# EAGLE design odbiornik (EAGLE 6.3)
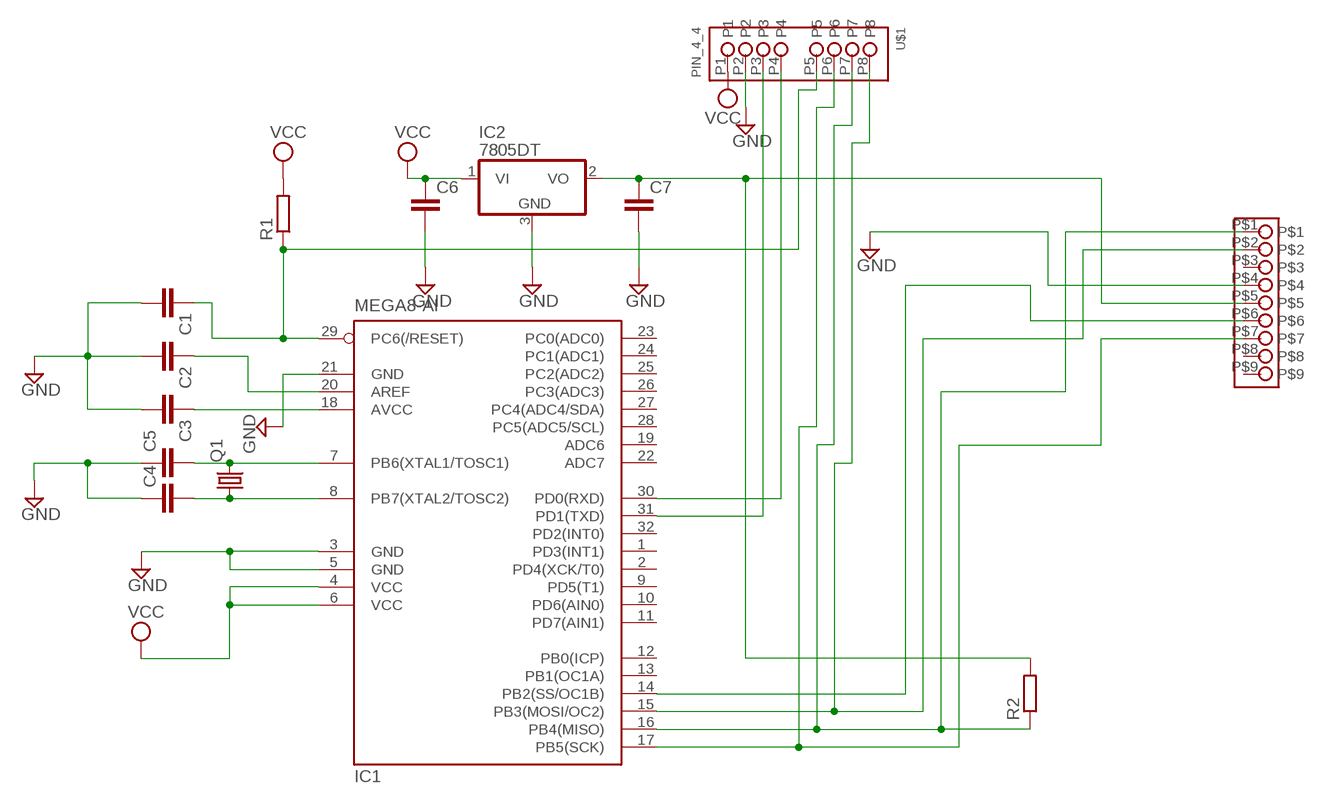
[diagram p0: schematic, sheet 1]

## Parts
C1  C-EUC0805  [C0805]
C2  C-EUC0805  [C0805]
C3  C-EUC0805  [C0805]
C4  C-EUC0805  [C0805]
C5  C-EUC0805  [C0805]
C6  C-EUC0805  [C0805]
C7  C-EUC0805  [C0805]
IC1  MEGA8-AI  [TQFP32-08]
IC2  7805DT  [TO252]
Q1  CRYSTALHC49UP  [HC49UP]
R1  R-EU_M0805  [M0805]
R2  R-EU_R0805  [R0805]
U$1  PIN_4_4  [PIN_4_4]
U$2  PIN_4MM  [PIN_4MM]

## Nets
GND: C1.2 C2.2 C3.2 C4.1 C5.1 C6.2 C7.2 IC1.3(GND) IC1.5(GND) IC1.21(GND) IC2.3(GND) U$1.P2 U$2.P$4
N$1: C3.1 IC1.18(AVCC)
N$2: C2.1 IC1.20(AREF)
N$3: C1.1 IC1.29(PC6(/RESET)) R1.1 U$1.P5
N$4: C5.2 IC1.7(PB6(XTAL1/TOSC1)) Q1.2
N$5: C4.2 IC1.8(PB7(XTAL2/TOSC2)) Q1.1
N$6: IC1.17(PB5(SCK)) U$1.P6 U$2.P$7
N$7: IC1.16(PB4(MISO)) R2.1 U$1.P7 U$2.P$1
N$8: IC1.15(PB3(MOSI/OC2)) U$1.P8 U$2.P$2
N$9: IC1.14(PB2(SS/OC1B)) U$2.P$6
N$10: C7.1 IC2.2(VO) R2.2 U$2.P$5
N$11: IC1.31(PD1(TXD)) U$1.P3
N$12: IC1.30(PD0(RXD)) U$1.P4
VCC: C6.1 IC1.4(VCC) IC1.6(VCC) IC2.1(VI) R1.2 U$1.P1
Unconnected: IC1.1(PD3(INT1)) IC1.2(PD4(XCK/T0)) IC1.9(PD5(T1)) IC1.10(PD6(AIN0)) IC1.11(PD7(AIN1)) IC1.12(PB0(ICP)) IC1.13(PB1(OC1A)) IC1.19(ADC6) IC1.22(ADC7) IC1.23(PC0(ADC0)) IC1.24(PC1(ADC1)) IC1.25(PC2(ADC2)) IC1.26(PC3(ADC3)) IC1.27(PC4(ADC4/SDA)) IC1.28(PC5(ADC5/SCL)) IC1.32(PD2(INT0)) U$2.P$3 U$2.P$8 U$2.P$9

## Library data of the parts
C1-C7 = rcl:C-EU: CAPACITOR, European symbol
IC1 = atmel:MEGA8: MICROCONTROLLER 8 Kbytes FLASH, 1 kbytes SRAM, 512 bytes EEPROM, USART, 6-channel 10 bit ADC, 2-channel 8 bit ADC Pin compatible with Atmega48, ATMega88, ATMega168 Source: avr.lbr
IC2 = linear:78*: Positive VOLTAGE REGULATOR Source: http://cache.national.com/ds/LM/LM78L05.pdf http://www.fairchildsemi.com/ds/LM/LM7805.pdf
Q1 = crystal:CRYSTAL: CRYSTAL
R1 R2 = rcl:R-EU_: RESISTOR, European symbol
U$1 = pin_4_4:PIN_4_4
U$2 = pin_4mm:PIN_4MM

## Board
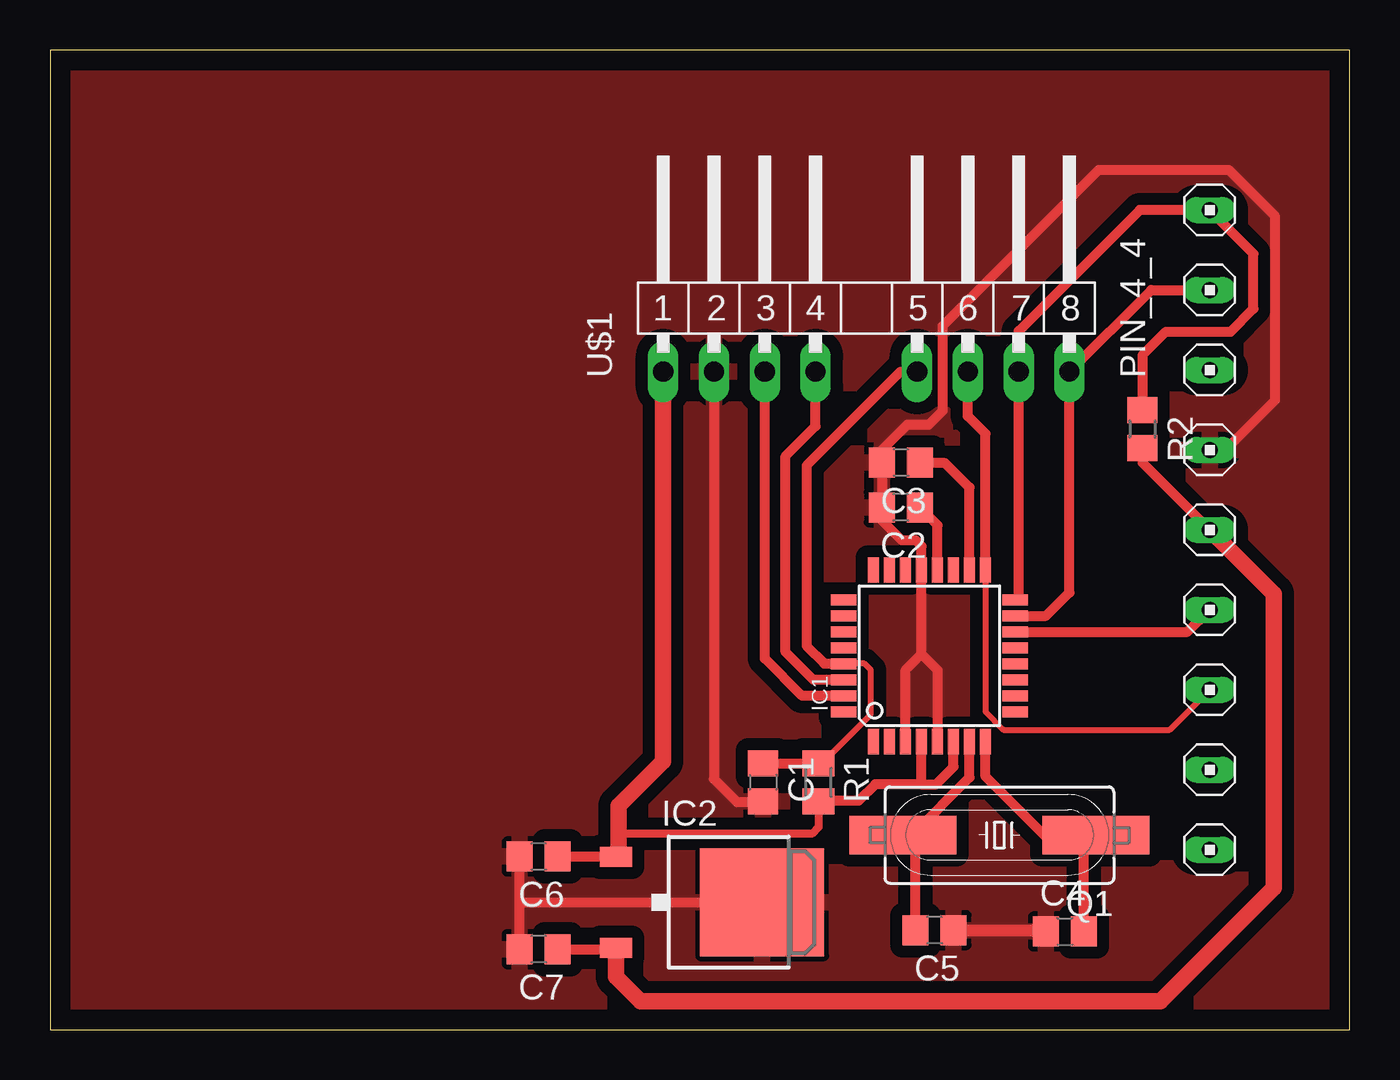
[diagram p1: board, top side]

Size 65 x 49.02 mm. Coordinates in mm from the lower left corner, seen from the top.
Outline: 0,0 65,0 65,49.02 0,49.02 0,0
Copper layers (1*16): Top 0.035mm / dielectric 1.5mm / Bottom 0.035mm
Design rules "default": minimum track width 10mil, minimum drill 24mil, track to track 8mil, track to pad 8mil, pad to pad 8mil, via to via 8mil, smd to smd 8mil, copper to edge 40mil, drill to drill 8mil, minimum pad ring 10mil, minimum via ring 8mil, stop-mask expansion 4mil, vias tented up to drill 0mil, thermal gap 10mil

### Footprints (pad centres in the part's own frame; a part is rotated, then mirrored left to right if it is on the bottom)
C0805 = smd 1.3 x 1.5: 1 -0.95,0; 2 0.95,0
TQFP32-08 = smd 1.27 x 0.559: 1 -4.293,2.8; 2 -4.293,2; 3 -4.293,1.2; 4 -4.293,0.4; 5 -4.293,-0.4; 6 -4.293,-1.2; 7 -4.293,-2; 8 -4.293,-2.8; 17 4.293,-2.8; 18 4.293,-2; 19 4.293,-1.2; 20 4.293,-0.4; 21 4.293,0.4; 22 4.293,1.2; 23 4.293,2; 24 4.293,2.8 | smd 0.559 x 1.27: 9 -2.8,-4.293; 10 -2,-4.293; 11 -1.2,-4.293; 12 -0.4,-4.293; 13 0.4,-4.293; 14 1.2,-4.293; 15 2,-4.293; 16 2.8,-4.293; 25 2.8,4.293; 26 2,4.293; 27 1.2,4.293; 28 0.4,4.293; 29 -0.4,4.293; 30 -1.2,4.293; 31 -2,4.293; 32 -2.8,4.293
TO252 = smd 1 x 1.6: 1 -2.28,-4.8; 2 2.28,-4.8 | smd 5.4 x 6.2: 3 0,2.5
HC49UP = smd 5.334 x 1.93: 1 -4.826,0; 2 4.826,0
M0805 = smd 1.3 x 1.6: 1 -0.95,0; 2 0.95,0
R0805 = smd 1.3 x 1.5: 1 -0.95,0; 2 0.95,0
PIN_4_4 = drill 1.016 long: P1 -10.16,0.318; P2 -7.62,0.318; P3 -5.08,0.318; P4 -2.54,0.318; P5 2.54,0.318; P6 5.08,0.318; P7 7.62,0.318; P8 10.16,0.318
PIN_4MM = drill 0.8 long: P$1 -16,0; P$2 -12,0; P$3 -8,0; P$4 -4,0; P$5 0,0; P$6 4,0; P$7 8,0; P$8 12,0; P$9 16,0

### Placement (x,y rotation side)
C1  35.67,12.39 270 top
C2  42.55,26.14 180 top
C3  42.57,28.37 180 top
C4  50.77,4.93 0 top
C5  44.25,4.98 180 top
C6  24.45,8.67 180 top
C7  24.45,4.03 180 top
IC1  43.99,18.71 90 top
IC2  33.11,6.38 270 top
Q1  47.49,9.74 180 top
R1  38.44,12.39 270 top
R2  54.64,30.06 270 top
U$1  40.83,32.61 0 top
U$2  58,25.02 270 top

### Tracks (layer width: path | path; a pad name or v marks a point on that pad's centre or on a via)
GND
  Top 0.508: IC1.3 42.79,17.99 43.59,18.79 | 43.59,18.79 IC1.21 43.59,24.2 43.31,24.48 42.61,24.48 41.53,25.56 41.53,26.06 C2.2 41.62,26.16 C3.2 41.59,28.4 41.59,28.99 42.86,30.26 43.94,30.26 44.64,30.96 44.64,35.21 52.45,43.02 58.96,43.02 61.28,40.7 61.28,31.5 58.8,29.02 U$2.P$4 | IC1.5 44.39,17.99 43.59,18.79 | C7.2 23.5,6.32 | 23.5,6.32 C6.2 | 23.5,6.32 23.56,6.38 IC2.3 | C1.2 35.63,11.4 34.35,11.4 33.21,12.54 U$1.P2
  Top 0.61: C5.1 49.76,4.98 C4.1
  pour Top (isolate 0.61): -0.32,49.72 -0.32,-0.51 65.47,-0.51 65.47,49.72
N$1
  Top 0.508: IC1.18 45.99,27.13 44.77,28.35 43.99,28.35 C3.1
N$2
  Top 0.508: IC1.20 44.39,25.25 C2.1
N$3
  Top 0.305: 38.61,13.34 41.05,15.78 41.05,18 40.73,18.32 39.71,18.32
  Top 0.406: R1.1 38.61,13.34 | 39.71,18.32 IC1.29
  Top 0.508: C1.1 R1.1 | IC1.29 39.69,18.32 38.73,18.32 37.85,19.21 37.85,28.23 42.55,32.93 U$1.P5
N$4
  Top 0.508: 43.18,9.81 42.73,9.81 Q1.2 | 42.85,9.48 43.18,9.81 | IC1.7 45.99,12.62 43.18,9.81 | C5.2 43.3,9.69 43.18,9.81
N$5
  Top 0.508: 52.17,9.6 Q1.1 52.19,9.62 51.31,9.62 | IC1.8 46.79,12.68 49.85,9.62 51.31,9.62 | C4.2 51.72,9.21 51.31,9.62
N$6
  Top 0.305: IC1.17 46.79,15.92 47.69,15.02 56,15.02 U$2.P$7
  Top 0.508: IC1.17 46.79,29.82 45.91,30.7 U$1.P6
N$7
  Top 0.508: IC1.16 48.45,21.68 U$1.P7 48.45,34.96 54.51,41.02 U$2.P$1 60.2,38.82 60.2,36.07 59.05,34.92 55.82,34.92 54.64,33.75 R2.1
N$8
  Top 0.508: IC1.15 49.82,20.71 50.99,21.88 U$1.P8 55.08,37.02 U$2.P$2
N$9
  Top 0.508: IC1.14 56.89,19.91 U$2.P$6
N$10
  Top 0.508: C7.1 28.24,4.03 IC2.2 | R2.2 54.64,28.38 U$2.P$5
  Top 0.813: IC2.2 28.31,2.64 29.53,1.42 55.53,1.42 61.21,7.11 61.21,21.8 U$2.P$5
N$11
  Top 0.508: IC1.31 37.62,16.71 35.75,18.57 U$1.P3
N$12
  Top 0.508: IC1.30 38.18,17.51 36.8,18.89 36.8,28.7 38.29,30.2 U$1.P4
VCC
  Top 0.406: R1.2 38.44,10.15 38.1,9.81 28.7,9.81 28.45,9.56
  Top 0.508: IC1.6 45.19,13.15 44.32,12.29 43.56,12.29 | IC1.4 43.59,12.32 43.56,12.29 | C6.1 IC2.1 28.32,8.67 | 43.56,12.29 41.27,12.29 40.45,11.46 38.46,11.46 R1.2
  Top 0.813: U$1.P1 30.67,13.43 28.45,11.21 28.45,9.56 28.45,8.8 IC2.1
